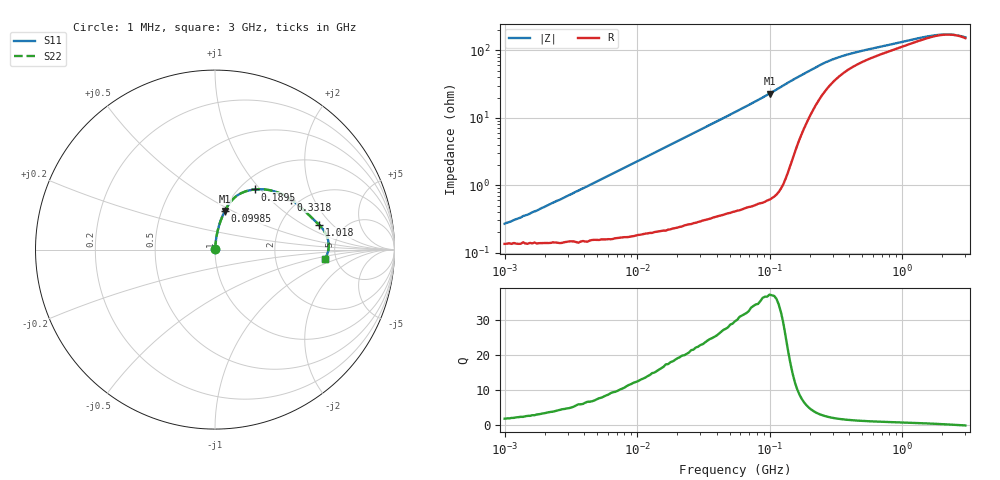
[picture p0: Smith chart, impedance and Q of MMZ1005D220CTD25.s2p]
! S-Parameter Data Generated by TDK Corporation
! Copyright(C) 2025 TDK Corporation.
! All Rights Reserved.
! TDK P/N: MMZ1005D220CTD25 (Chip Bead)
! Property: |Z|=22ohm at 100MHz
! Size(LxWxT): 1x0.5x0.5mm
! Model Type: s2p (Touchstone File Format Version 1.0)
! Frequency: DC=Yes Start=1MHz Stop=3000MHz 202points Log-sweep
! Model Generated on Feb. 6, 2025
! Terms and conditions regarding TDK Simulation Models:
! 1)This simulation model is being provided solely for informational
!  purposes. Please refer to the specifications of the products in
!  terms of detailed characteristics of such products.
! 2)In no event shall TDK Corporation of any of its subsidiaries be
!  liable for any loss or damage arising, directly or indirectly,
!  from any information contained in this simulation model, including,
!  but not limited to loss or damages arising from any inaccuracies,
!  omissions or errors in connection with such information.
! 3)Any and all copyrights on this simulation model are owned by
!  TDK Corporation.  Duplication or redistribution of this simulation
!  model without prior written permission from TDK Corporation
!  is prohibited.
! 4)This simulation model is subject to any modification or change
!  without any prior notice.
! 5)Neither TDK Corporation nor any of its subsidiaries shall make any
!  warranty, express or implied, including but not limited to the
!  correctness, implied warranties of merchantability and fitness for
!  a particular purpose with respect to this simulation models.
! 6)The use of this simulation model shall be deemed to have consented
!  to the terms and conditions hereof.
! Port Assignments:
!  1 ---@@@--- 2
! Applicable Conditions:
!  Temperature = 25 degC
!  DC Bias Current = 0 A
!  Small Signal Operation
# Hz S MA R 50
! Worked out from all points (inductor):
!   201 points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, 1 MHz to 3 GHz, reference 50 ohm
!   read as one part in series: L = 36.4 nH near 1.823 MHz
!   highest Q = 37 at 99.85 MHz (marker M1), where L = 36.5 nH
!   self-resonance near 2.347 GHz
!   S11 on the Smith chart (normalised r, x): 1 MHz: 1.00, +0.00; 99.85 MHz: 1.01, +0.46; 189.5 MHz: 1.17, +0.93; 331.8 MHz: 1.81, +1.36; 1.018 GHz: 3.31, +1.41; 3 GHz: 4.05, -0.72
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1000000  0.002681 59.7  0.9987 -0.1  0.9987 -0.1  0.002681 59.7
1751453  0.004195 70.8  0.9986 -0.2  0.9986 -0.2  0.004195 70.8
3900413  0.008974 80.0  0.9985 -0.5  0.9985 -0.5  0.008974 80.0
1.461624e7  0.03269 84.5  0.9974 -1.9  0.9974 -1.9  0.03269 84.5
3.00453e7  0.06632 83.7  0.9949 -3.8  0.9949 -3.8  0.06632 83.7
5.477226e7  0.1202 81.2  0.9887 -6.9  0.9887 -6.9  0.1202 81.2
7.544761e7  0.1659 78.8  0.9813 -9.5  0.9813 -9.5  0.1659 78.8
9.984923e7  0.2219 75.7  0.9692 -12.8  0.9692 -12.8  0.2219 75.7
1.171891e8  0.2637 73.1  0.957 -15.3  0.957 -15.3  0.2637 73.1
1.375402e8  0.3117 69.2  0.9358 -18.1  0.9358 -18.1  0.3117 69.2
1.614254e8  0.358 63.5  0.8994 -20.9  0.8994 -20.9  0.358 63.5
1.894586e8  0.4013 56.6  0.8482 -23.3  0.8482 -23.3  0.4013 56.6
2.136344e8  0.4323 51.0  0.8014 -24.8  0.8014 -24.8  0.4323 51.0
2.716345e8  0.4812 40.3  0.7053 -26.2  0.7053 -26.2  0.4812 40.3
3.318279e8  0.5077 33.3  0.6397 -25.8  0.6397 -25.8  0.5077 33.3
4.75755e8  0.5392 24.6  0.5568 -23.8  0.5568 -23.8  0.5392 24.6
8.005644e8  0.5777 16.5  0.4753 -20.2  0.4753 -20.2  0.5777 16.5
1.017911e9  0.5968 13.3  0.4413 -18.2  0.4413 -18.2  0.5968 13.3
1.581072e9  0.627 7.0  0.3853 -11.4  0.3853 -11.4  0.627 7.0
2.01032e9  0.634 2.9  0.3682 -5.0  0.3682 -5.0  0.634 2.9
2.455801e9  0.6303 -0.9  0.3699 1.5  0.3699 1.5  0.6303 -0.9
3e9  0.6139 -5.1  0.3925 8.1  0.3925 8.1  0.6139 -5.1
